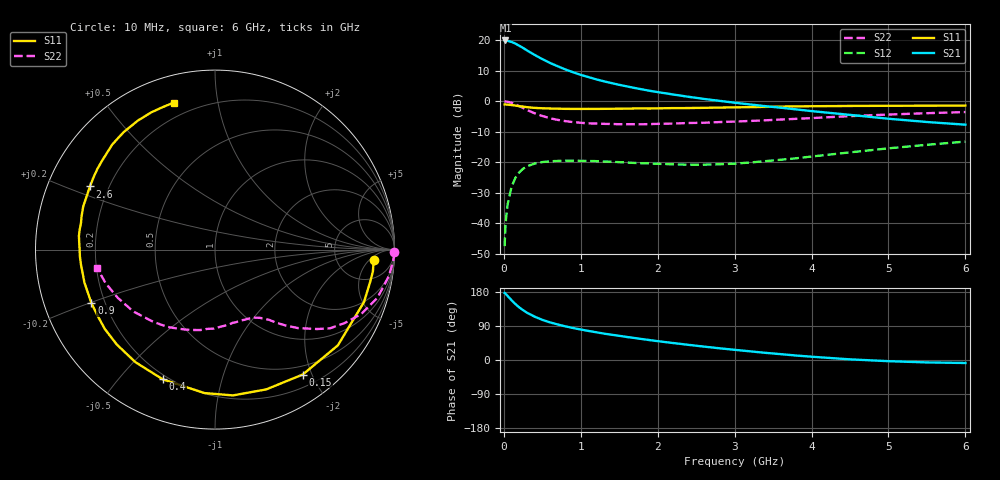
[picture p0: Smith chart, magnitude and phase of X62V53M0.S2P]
! SIEMENS Small Signal Semiconductors
! BFP193W
! Si NPN RF Bipolar Junction Transistor in SOT343
! VCE = 2.5 V  IC = 3 mA
! Common Emitter S-Parameters:  April 1994
# GHz  S  MA  R  50
!  f  S11  S21  S12  S22
! GHz  MAG  ANG  MAG  ANG  MAG  ANG  MAG  ANG
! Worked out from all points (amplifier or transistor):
!   40 points, 10 MHz to 6 GHz, reference 50 ohm
!   highest |S21| = 19.9 dB at 20 MHz (marker M1)
!   |S21| within 3 dB of that: start of sweep to 284.2 MHz
!   unconditionally stable (mu >= 1): 1.901 GHz to 4.609 GHz
!   at 200 MHz: K = 0.11, MSG = 20.8 dB, |S12| = -23.3 dB
!   at 1.5 GHz: K = 0.79, MSG = 12.7 dB, |S12| = -20.0 dB
!   at 6 GHz: K = 0.95, MSG = 2.8 dB, |S12| = -13.2 dB
!   S11 on the Smith chart (normalised r, x): 10 MHz: 13, -7; 150 MHz: 0.37, -1.87; 400 MHz: 0.18, -0.66; 900 MHz: 0.15, -0.20; 2.6 GHz: 0.13, +0.23; 6 GHz: 0.13, +0.75
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0.01  0.8861 -3.9  9.868 176.9  0.0042 89.4  1 -0.9
0.02  0.8881 -7.9  9.942 175.4  0.0083 84.9  0.9949 -3.7
0.05  0.88 -19.4  9.81 168.7  0.0207 79.3  0.9797 -8.7
0.1  0.8679 -37.9  9.396 157.8  0.0393 69.9  0.9442 -16.5
0.15  0.8507 -54.9  8.839 147.7  0.0556 61.1  0.8908 -23.7
0.2  0.8295 -69.9  8.145 138.9  0.0682 53.4  0.8317 -29.4
0.25  0.8185 -83.0  7.502 131.5  0.0782 47.0  0.7764 -34.4
0.3  0.8014 -94.2  6.834 124.9  0.0857 41.9  0.7204 -37.9
0.4  0.7793 -111.9  5.76 114.4  0.095 33.5  0.635 -43.5
0.5  0.768 -125.3  4.918 106.0  0.1006 27.7  0.5736 -47.3
0.6  0.761 -136.0  4.252 99.3  0.1035 23.2  0.5273 -50.3
0.7  0.7566 -144.2  3.753 93.8  0.1051 20.3  0.4953 -52.3
0.9  0.75 -156.7  2.994 84.4  0.1062 15.6  0.4554 -56.6
1.1  0.7504 -165.9  2.492 76.7  0.105 12.8  0.4342 -60.6
1.3  0.7516 -173.7  2.128 69.7  0.103 11.1  0.4261 -65.0
1.6  0.7577 176.9  1.754 60.7  0.099 11.1  0.4206 -71.5
2.2  0.7726 161.9  1.292 44.8  0.0924 15.5  0.4307 -85.9
2.6  0.7806 153.2  1.094 35.4  0.0913 21.8  0.4442 -95.8
3.2  0.8014 141.4  0.887 22.9  0.099 31.7  0.4755 -110.5
4.5  0.8375 120.8  0.598 1.7  0.1452 42.0  0.5709 -142.8
5.5  0.8453 110.5  0.457 -6.4  0.1932 39.8  0.6376 -163.0
6  0.8507 105.7  0.413 -7.9  0.2181 37.5  0.6654 -171.1
